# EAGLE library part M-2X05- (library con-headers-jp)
MALE HEADER
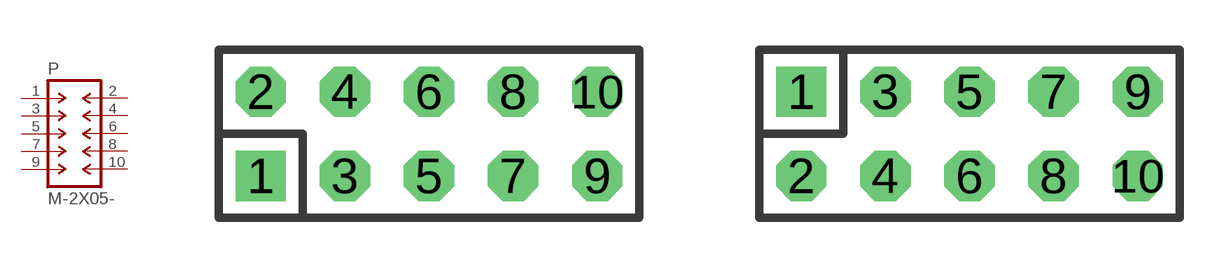
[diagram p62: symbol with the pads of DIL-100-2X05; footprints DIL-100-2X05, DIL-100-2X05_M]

Designator prefix P

## M-2X05-DIL-100  [DIL-100-2X05]
1  1  pas
2  2  pas
3  3  pas
4  4  pas
5  5  pas
6  6  pas
7  7  pas
8  8  pas
9  9  pas
10  10  pas

## M-2X05-DIL-100_M  [DIL-100-2X05_M]
Pads as for DIL-100-2X05

## M-2X05-DIL-2MM  [DIL-2MM-2X05]
Pads as for DIL-100-2X05

## M-2X05-DIL-2MM_M  [DIL-2MM-2X05_M]
Pads as for DIL-100-2X05

## M-2X05-87759  [87759-10]
Pads as for DIL-100-2X05

## M-2X05-87759_M  [87759-10_M]
Pads as for DIL-100-2X05

## Footprint DIL-100-2X05 (pad centres in mm)
PIN HEADER - 0.1"
drill 1.016 square: 1 -5.08,-1.27
drill 1.016 octagon: 2 -5.08,1.27; 3 -2.54,-1.27; 4 -2.54,1.27; 5 0,-1.27; 6 0,1.27; 7 2.54,-1.27; 8 2.54,1.27; 9 5.08,-1.27; 10 5.08,1.27

## Footprint DIL-100-2X05_M (pad centres in mm)
PIN HEADER - MIRRORED 0.1"
drill 1.016 square: 1 -5.08,1.27
drill 1.016 octagon: 2 -5.08,-1.27; 3 -2.54,1.27; 4 -2.54,-1.27; 5 0,1.27; 6 0,-1.27; 7 2.54,1.27; 8 2.54,-1.27; 9 5.08,1.27; 10 5.08,-1.27

## Footprint DIL-2MM-2X05 (pad centres in mm)
PIN HEADER - 2MM"
drill 0.711 square: 1 -4,-1
drill 0.711: 2 -4,1; 3 -2,-1; 4 -2,1; 5 0,-1; 6 0,1; 7 2,-1; 8 2,1; 9 4,-1; 10 4,1

## Footprint DIL-2MM-2X05_M (pad centres in mm)
PIN HEADER - MIRRORED 2MM
drill 0.711 square: 1 -4,1
drill 0.711: 2 -4,-1; 3 -2,1; 4 -2,-1; 5 0,1; 6 0,-1; 7 2,1; 8 2,-1; 9 4,1; 10 4,-1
